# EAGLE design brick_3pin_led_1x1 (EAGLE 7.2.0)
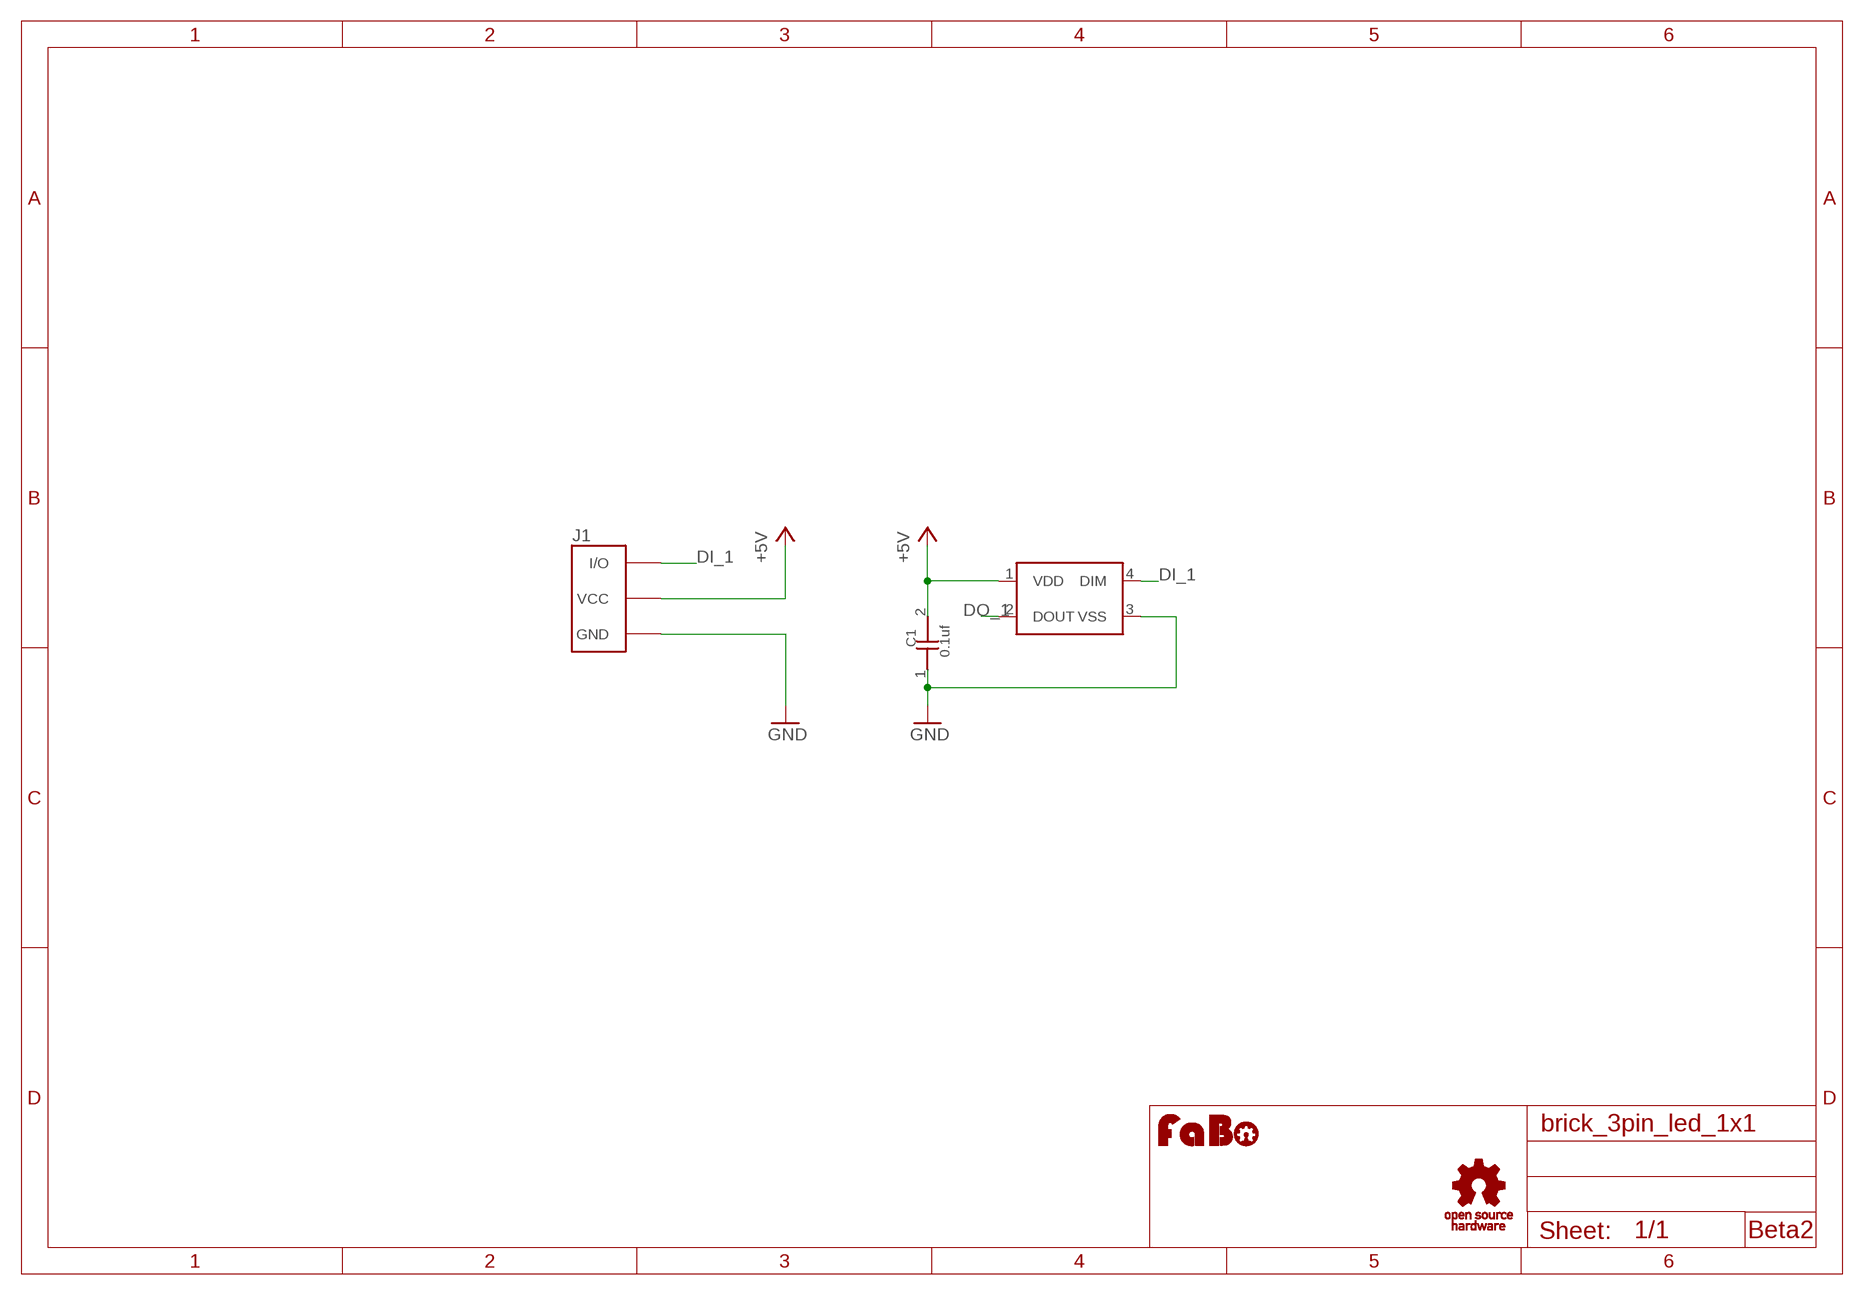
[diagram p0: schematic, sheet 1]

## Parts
C1  0.1uf  CAPACITOR0603  [0603]
J1  BRICK_3PIN_NORMAL  [BRICK_3PIN]
LED1  WS2818B  [WS2818B]
U$4  LOGO_FABO-M  [LOGO_FABO_M]
U$5  LOGO_OSHW_T-M  [LOGO_OSHW_T_M]

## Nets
+5V: C1.2 J1.VCC LED1.1(VDD)
DI_1: J1.IN/OUT(I/O) LED1.4(DIM)
DO_1: LED1.2(DOUT)
GND: C1.1 J1.GND LED1.3(VSS)

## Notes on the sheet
- Beta2

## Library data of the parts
C1 = GClue-Capacitor:CAPACITOR
J1 = GClue:BRICK_3PIN: FaBo Brick 3pin
LED1 = GClue-LED:WS2818B
U$4 = FaBo:LOGO_FABO
U$5 = GClue:LOGO_OSHW_T

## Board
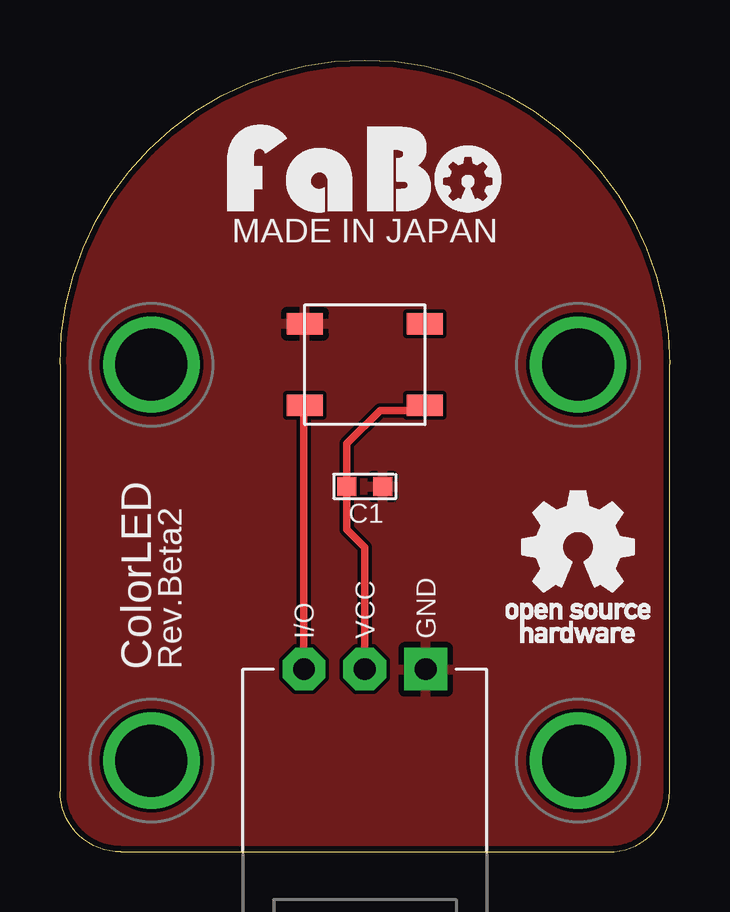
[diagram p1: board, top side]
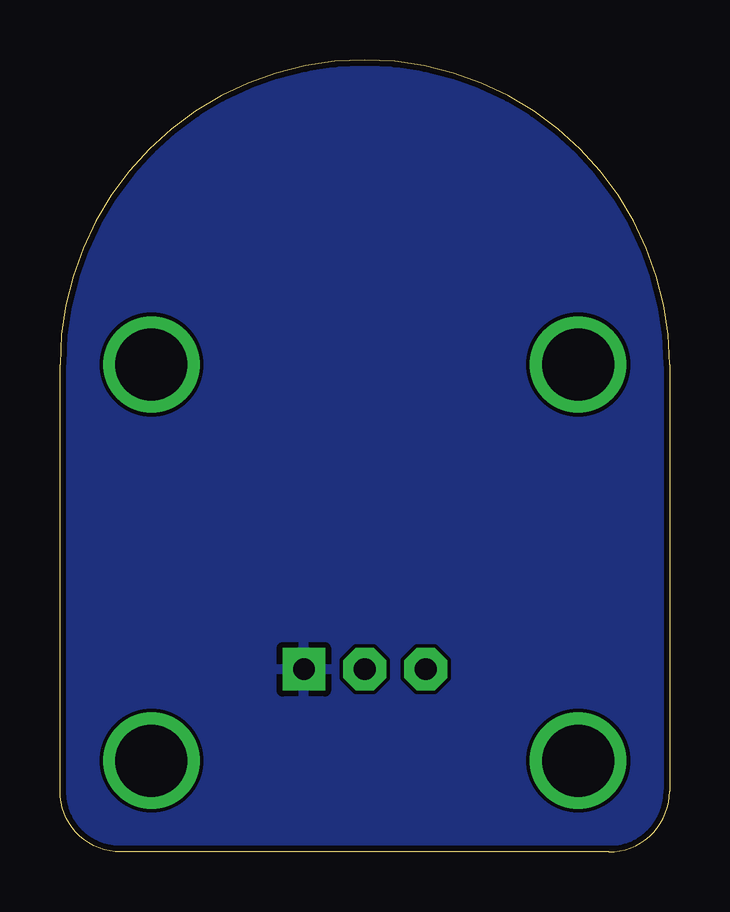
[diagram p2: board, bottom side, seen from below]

Size 25.4 x 33.02 mm. Coordinates in mm from the lower left corner, seen from the top.
Copper layers (1*16): Top 0.035mm / dielectric 1.5mm / Bottom 0.035mm
Design rules "Elecrow_2-layer_eagle_rule": minimum track width 6mil, minimum drill 12mil, track to track 6mil, track to pad 6mil, pad to pad 6mil, via to via 6mil, smd to smd 0mil, copper to edge 10mil, drill to drill 10mil, minimum pad ring 10mil, minimum via ring 6mil, stop-mask expansion 2mil, vias tented up to drill 100mil, thermal gap 10mil

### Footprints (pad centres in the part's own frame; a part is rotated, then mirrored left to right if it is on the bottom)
0603 = smd 0.8 x 0.8: 1 -0.75,0; 2 0.75,0
BRICK_3PIN = drill 0.9 pad 1.778 square: GND 2.54,-8.89 | drill 0.9 pad 1.778 octagon: IN/OUT -2.54,-8.89; VCC 0,-8.89 | drill 3 pad 3.81: P$5 -8.89,3.81; P$6 8.89,3.81; P$7 -8.89,-12.7; P$8 8.89,-12.7
WS2818B = smd 1.5 x 0.9: 1 -2.5,1.7; 2 -2.5,-1.7; 3 2.5,-1.7; 4 2.5,1.7

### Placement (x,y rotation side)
C1  12.7,15.24 180 top
J1  12.7,16.51 0 top
LED1  12.7,20.32 180 top
U$4  12.7,26.67 0 top
U$5  21.59,12.7 0 top

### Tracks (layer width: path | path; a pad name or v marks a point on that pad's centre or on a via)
+5V
  Top 0.305: J1.VCC 12.7,12.7 11.95,13.45 C1.2 11.95,17.03 13.34,18.41 14.99,18.41 LED1.1
DI_1
  Top 0.305: LED1.4 10.16,18.62 J1.IN/OUT
GND
  pour Bottom: -1.27,-1.27 26.67,-1.27 26.67,34.29 -1.27,34.29
  pour Top: -1.27,-1.27 26.67,-1.27 26.67,34.29 -1.27,34.29

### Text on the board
tPlace: MADE IN JAPAN | ColorLED | Rev.Beta2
